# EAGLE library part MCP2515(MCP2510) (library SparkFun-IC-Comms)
CAN controller with SPI interface The MCP2515 controller supercedes the MCP2510 while addressing all errata associated with it. The two devices are pin compatible, either can be used with this device. 18-pin package SOIC Simple SPI interface to any MCU. One-shot mode ensures message transmission is attempted only once Databyte filtering Start-of-Frame (SOF) output Low-power CMOS Technology Datasheet SparkFun Products CAN-BUS Shield (DEV-13262)
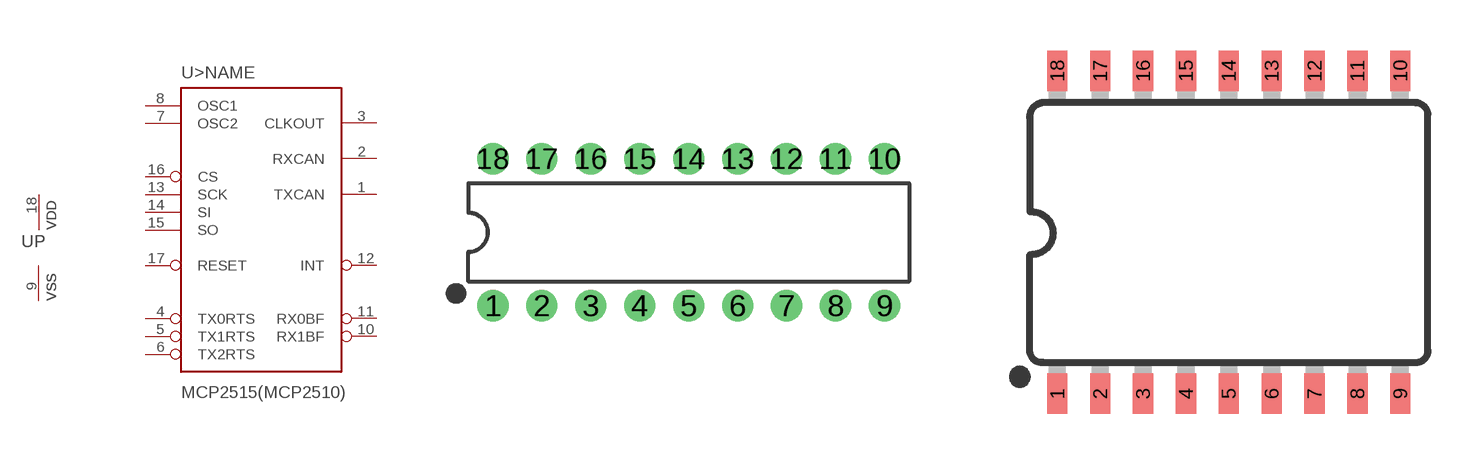
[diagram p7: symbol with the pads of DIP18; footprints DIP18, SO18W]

Designator prefix U; gates >NAME=MCP2510 P=PWRN-1

## MCP2515(MCP2510)P (PROD_ID: NA-XXXXX; VALUE: MCP2515)  [DIP18]
1  >NAME:TXCAN  out
2  >NAME:RXCAN  in
3  >NAME:CLKOUT  out
4  >NAME:TX0RTS  in
5  >NAME:TX1RTS  in
6  >NAME:TX2RTS  in
7  >NAME:OSC2  out
8  >NAME:OSC1  in
9  P:VSS  pwr
10  >NAME:RX1BF  out
11  >NAME:RX0BF  out
12  >NAME:INT  out
13  >NAME:SCK  in
14  >NAME:SI  in
15  >NAME:SO  out
16  >NAME:CS  in
17  >NAME:RESET  in
18  P:VDD  pwr

## MCP2515(MCP2510)SO (PROD_ID: IC-09906; VALUE: MCP2515)  [SO18W]
Pads as for DIP18

## Footprint DIP18 (pad centres in mm)
Dual In Line Package -18 Specifications: Pin count:18 Example device(s): MCP2515(MCP2510)
drill 0.813 pad 1.626: 1 -10.16,-3.81; 2 -7.62,-3.81; 3 -5.08,-3.81; 4 -2.54,-3.81; 5 0,-3.81; 6 2.54,-3.81; 7 5.08,-3.81; 8 7.62,-3.81; 9 10.16,-3.81; 10 10.16,3.81; 11 7.62,3.81; 12 5.08,3.81; 13 2.54,3.81; 14 0,3.81; 15 -2.54,3.81; 16 -5.08,3.81; 17 -7.62,3.81; 18 -10.16,3.81

## Footprint SO18W (pad centres in mm)
Small Outline Wide Plastic Gull Wing SOIC, 0.3 inch width
smd 0.6 x 1.2: 1 -5.08,-4.788; 2 -3.81,-4.788; 3 -2.54,-4.788; 4 -1.27,-4.788; 5 0,-4.788; 6 1.27,-4.788; 7 2.54,-4.788; 8 3.81,-4.788; 9 5.08,-4.788; 10 5.08,4.788; 11 3.81,4.788; 12 2.54,4.788; 13 1.27,4.788; 14 0,4.788; 15 -1.27,4.788; 16 -2.54,4.788; 17 -3.81,4.788; 18 -5.08,4.788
